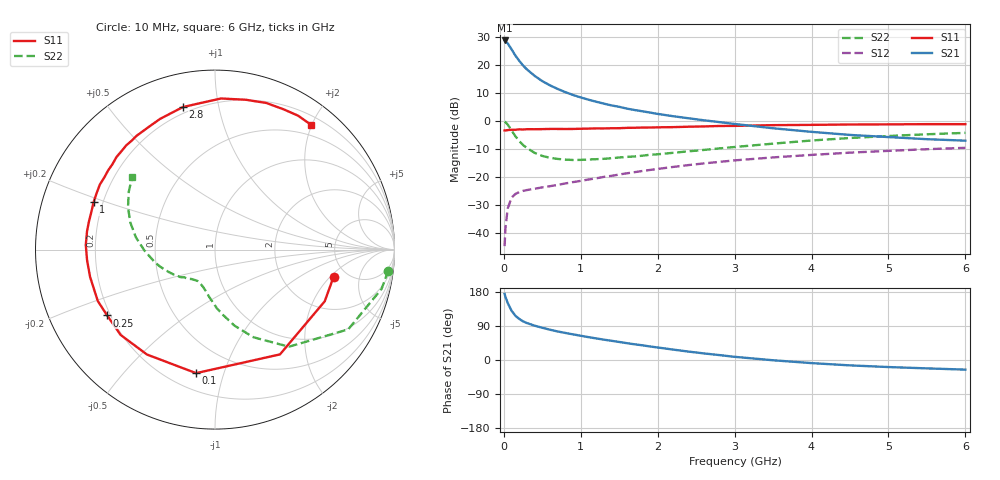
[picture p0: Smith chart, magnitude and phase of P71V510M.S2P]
! SIEMENS Small Signal Semiconductors
! BFP196
! Si NPN RF Bipolar Junction Transistor in SOT143
! VCE = 1.5 V  IC = 10 mA
! Common Emitter S-Parameters:  May  1996
# GHz  S  MA  R  50
!  f  S11  S21  S12  S22
! GHz  MAG  ANG  MAG  ANG  MAG  ANG  MAG  ANG
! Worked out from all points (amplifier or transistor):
!   36 points, 10 MHz to 6 GHz, reference 50 ohm
!   highest |S21| = 28.9 dB at 10 MHz (marker M1)
!   |S21| within 3 dB of that: start of sweep to 95.92 MHz
!   unconditionally stable (mu >= 1): 848.2 MHz to 3.368 GHz
!   at 250 MHz: K = 0.41, MSG = 22.5 dB, |S12| = -25.1 dB
!   at 1.4 GHz: K = 1.16, MAG = 10.2 dB, |S12| = -19.7 dB
!   at 6 GHz: K = 0.99, MSG = 1.3 dB, |S12| = -9.6 dB
!   S11 on the Smith chart (normalised r, x): 10 MHz: 3.90, -2.20; 100 MHz: 0.30, -0.81; 250 MHz: 0.19, -0.27; 1 GHz: 0.16, +0.18; 2.8 GHz: 0.17, +0.79; 6 GHz: 0.33, +1.98
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0.01  0.6778 -13.0  27.8 174.5  0.0057 84.5  0.9721 -6.9
0.02  0.6759 -25.2  27.05 167.1  0.0118 77.6  0.954 -13.2
0.05  0.687 -58.2  24.7 150.6  0.0269 64.8  0.8653 -30.9
0.1  0.6963 -98.7  19.29 130.1  0.0423 48.2  0.6801 -52.7
0.15  0.6968 -123.0  14.93 116.8  0.0492 39.4  0.5336 -66.3
0.2  0.7088 -137.9  12.02 108.3  0.0532 35.1  0.4378 -75.6
0.25  0.704 -148.6  9.879 102.0  0.0559 32.3  0.3705 -82.5
0.3  0.7131 -156.3  8.41 97.5  0.0578 31.6  0.3276 -88.1
0.4  0.7124 -167.7  6.453 90.6  0.061 31.5  0.2683 -96.5
0.5  0.7151 -175.1  5.186 85.0  0.0646 32.6  0.2365 -102.6
0.6  0.7203 178.0  4.353 79.9  0.0678 34.1  0.219 -107.5
0.7  0.7202 172.0  3.757 75.3  0.0715 35.6  0.209 -111.9
0.8  0.7196 167.6  3.29 71.4  0.076 37.4  0.2032 -115.6
1  0.726 158.7  2.644 64.0  0.0845 39.9  0.2009 -121.2
1.1  0.7306 154.6  2.412 60.3  0.0893 40.7  0.2038 -123.8
1.6  0.7533 136.7  1.667 44.4  0.1155 42.7  0.2271 -135.9
2.2  0.7763 118.7  1.219 27.5  0.1501 40.8  0.2689 -148.9
2.8  0.8138 102.7  0.956 13.0  0.1848 36.0  0.3223 -163.3
3.5  0.8426 87.7  0.741 -0.7  0.2225 28.5  0.3927 -179.1
4.5  0.8655 70.7  0.563 -14.2  0.2709 17.5  0.4955 162.2
5.5  0.8782 58.2  0.472 -22.1  0.3122 6.3  0.578 146.3
6  0.8774 52.5  0.444 -25.4  0.3306 0.2  0.6129 139.0
